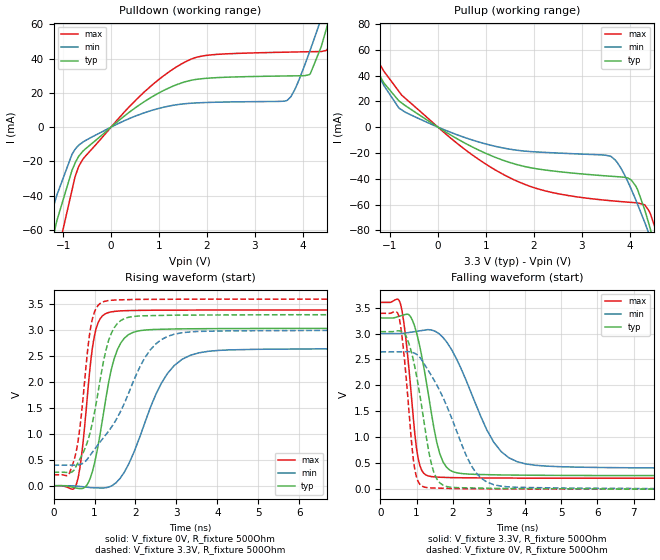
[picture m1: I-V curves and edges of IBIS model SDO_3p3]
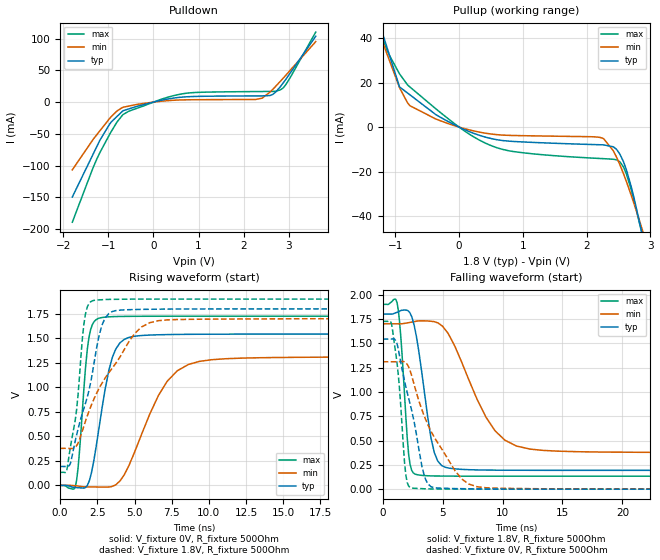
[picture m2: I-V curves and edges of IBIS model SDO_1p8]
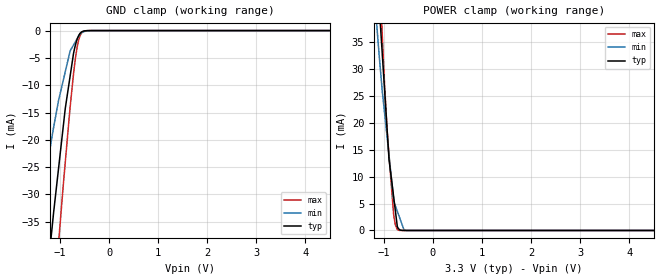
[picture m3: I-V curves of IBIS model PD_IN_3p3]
|Texas Instruments Incorporated
| INTEGRATED POWER AMPLIFIER MONITOR AND CONTROL SYSTEM
| Marketing part#   Digital Voltage Range   Package-type   #pins
| AMC7834   1.7V - 3.6V   PQFP   56
[IBIS Ver]   4.1
[File name]   amc7834.ibs
[File Rev]   1.0
[Date]   12/12/2013
[Source]
| Texas Instruments Incorporated.
| 12500 TI Blvd
| Dallas, TX -75243
[Notes]   Revision History:
| Rev 1.0: 12/12/2013
| - Initial version of the model
| - Model generated from simulations in TISPICE
| - C_comp although listed in numerical order of value are
|   obtained from varying PVT conditions. For PVT conditions for
|   each specific value refer the buffer description under
|   respective [Model]. IBIS model user is responsible for using
|   appropriate C_comp to simulate for Signal Integrity.
| - Model names with a trailing _1p8 contains the model for
|   1.8V operation.Model names with a trailing _3p3 contains the model
|   for 3.3V operation.
[Disclaimer]
| This model is designed as an aid for customers of Texas Instruments.
| TI and its licensors and suppliers make no warranties, either expressed
| or implied, with respect to this  model, including the warranties of
| merchantability or fitness for a particular purpose. The model is
| provided solely on an "as is" basis. The entire risk as to its quality
| and performance is with the customer.
[Copyright]
 (C) Copyright 2013 Texas Instruments Incorporated.All rights reserved.
|   Device
[Component]   AMC7834
[Manufacturer]   TI
[Package]
| variable   typ   min   max
R_pkg   0.079   0.031   0.106
L_pkg   1.073nH   0.648nH   1.372nH
C_pkg   0.150pF   0.128pF   0.230pF
[Pin]  signal_name   model_name   R_pin   L_pin   C_pin
1   DIGTEST/DAV   DAV   0.1053   1.37016nH   0.14918pF
2   ALARMOUT   GPIO   0.09756   1.25753nH   0.14389pF
3   SLEEP1   PD_IN   0.09216   1.17804nH   0.13837pF
4   SLEEP2   PD_IN   0.08922   1.13506nH   0.13484pF
5   RESETB   PD_IN   0.08788   1.1154nH   0.1331pF
6   DACTRIGB   PD_IN   0.08783   1.11459nH   0.13297pF
7   SCLK   PD_IN   0.08841   1.12318nH   0.13416pF
8   CSB   PD_IN   0.09063   1.15576nH   0.13641pF
9   SDI   PD_IN   0.09435   1.21049nH   0.1403pF
10   SDO   SDO   0.09971   1.28996nH   0.14738pF
11   DGND   GND   0.05243   0.93873nH   0.20017pF
12   IOVDD   POWER   0.03437   0.8265nH   0.22739pF
13   DVDD   POWER   0.03123   0.7166nH   0.21314pF
14   AVCC   POWER   0.04716   0.85425nH   0.17448pF
15   AUXDAC1   NC   0.10508   1.3668nH   0.15013pF
16   AUXDAC2   NC   0.09226   1.17816nH   0.1419pF
17   AGND1   GND   0.04621   0.74677nH   0.18488pF
18   AUXDACC3   NC   0.09212   1.1763nH   0.13877pF
19   AUXDACC4   NC   0.08893   1.12891nH   0.13535pF
20   REFIN   NC   0.08344   1.04761nH   0.13155pF
21   REFOUT   NC   0.07963   0.99042nH   0.12761pF
22   AGND2   GND   0.04047   0.64779nH   0.1651pF
23   DAC1   NC   0.08054   1.00265nH   0.1287pF
24   DAC2   NC   0.08248   1.03019nH   0.13198pF
25   AVSS   GND   0.04579   0.82708nH   0.17866pF
26   AVDD1   POWER   0.03183   0.772nH   0.20696pF
27   DAC3   NC   0.09598   1.22739nH   0.14561pF
28   DAC4   NC   0.10574   1.36956nH   0.14859pF
29   VCLAMP2   NC   0.09234   1.17055nH   0.13553pF
30   VCLAMP1   NC   0.08526   1.0683nH   0.13067pF
31   SENSE4-   NC   0.09275   1.179nH   0.13987pF
32   SENSE4+   NC   0.08261   1.02944nH   0.13079pF
33   SENSE3-   NC   0.08268   1.03069nH   0.13044pF
34   SENSE3+   NC   0.08044   0.9979nH   0.12812pF
35   AGND3   GND   0.04051   0.67363nH   0.15767pF
36   SENSE2-   NC   0.08032   0.99598nH   0.12906pF
37   SENSE2+   NC   0.08312   1.03711nH   0.13092pF
38   SENSE1-   NC   0.08304   1.0359nH   0.13159pF
39   SENSE1+   NC   0.0936   1.19177nH   0.14134pF
40   PA_ON   NC   0.09387   1.19554nH   0.14036pF
41   PAVDD   POWER   0.04917   0.87072nH   0.18625pF
42   REF_ADC/CMP   NC   0.0493   0.89668nH   0.17897pF
43   AGND4   GND   0.05376   0.99104nH   0.19612pF
44   AVDD2   POWER   0.03647   0.9263nH   0.23006pF
45   ADC4   NC   0.1057   1.37162nH   0.15535pF
46   ADC3   NC   0.09734   1.24786nH   0.14443pF
47   ADC2   NC   0.09048   1.14719nH   0.13737pF
48   ADC1   NC   0.08561   1.0763nH   0.13075pF
49   D2-   NC   0.09926   1.27608nH   0.14506pF
50   D2+   NC   0.08838   1.11645nH   0.13873pF
51   D1-   NC   0.08306   1.04024nH   0.13298pF
52   D1+   NC   0.08517   1.07249nH   0.13199pF
53   GPIO4   GPIO   0.0862   1.08664nH   0.13088pF
54   GPIO3   GPIO   0.08789   1.11204nH   0.13416pF
55   GPIO2   GPIO   0.09165   1.16832nH   0.13799pF
56   GPIO1   GPIO   0.09825   1.26426nH   0.14243pF
|   Model Selectors
[Model Selector]  SDO
SDO_3p3   SDO buffer in 3.3V power operation
SDO_1p8   SDO buffer in 1.8V power operation
[Model Selector]  PD_IN
PD_IN_3p3   PD_IN buffer in 3.3V power operation
PD_IN_1p8   PD_IN buffer in 1.8V power operation
[Model Selector]  GPIO
GPIO_3p3   GPIO buffer in 3.3V power operation
GPIO_1p8   GPIO buffer in 1.8V power operation
[Model Selector]  DAV
DAV_3p3   DAV buffer in 3.3V power operation
DAV_1p8   DAV buffer in 1.8V power operation
| Models and submodels in the file (8): SDO_3p3 (Output), SDO_1p8 (Output), PD_IN_3p3 (Input), PD_IN_1p8 (Input), GPIO_3p3 (I/O_open_drain), GPIO_1p8 (I/O_open_drain), DAV_3p3 (Output), DAV_1p8 (Output)
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|   Model
[Model]   SDO_3p3
Model_type   Output
Polarity   Non-Inverting
Vmeas = 1.65
Vref = 0
Cref = 1pF
Rref = 100000
|   typ   min   max
C_comp   3.353pF   3.015pF   3.780pF
[Voltage Range]   3.3   3   3.6
[Temperature Range]   27   125   -40
[Pullup Reference]   3.3   3   3.6
[Pulldown Reference]   0   0   0
[Power Clamp Reference]   3.3   3   3.6
[GND Clamp Reference]   0   0   0
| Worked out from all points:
|   slope of the pulldown table from 0 to 0.495 V, typ, clamps not added: 44.7 ohm
|   slope of the pullup table from 0 to 0.495 V, typ, clamps not added: 45 ohm
|   falling waveform, V_fixture 3.3V, R_fixture 500Ohm: 20-80 % time 466ps typ, 998ps min, 281ps max; typ from 3.3 V to 0.259 V
|   rising waveform, V_fixture 0V, R_fixture 500Ohm: 20-80 % time 426ps typ, 846ps min, 261ps max; typ from 0 V to 3.04 V
|   rising waveform, V_fixture 3.3V, R_fixture 500Ohm: 20-80 % time 470ps typ, 1.03ns min, 277ps max; typ from 0.259 V to 3.3 V
|   falling waveform, V_fixture 0V, R_fixture 500Ohm: 20-80 % time 444ps typ, 987ps min, 260ps max; typ from 3.04 V to 0 V
[Pulldown]
|   Voltage   I(typ)   I(min)   I(max)
-3.3V     -387.4mA   -282.5mA   -481.1mA
-1.359V   -84.44mA   -61.69mA   -110.2mA
-1.132V   -54.73mA   -39.76mA   -75.64mA
-587.4mV  -14.03mA   -8.722mA   -18.7mA
699.6mV   15.01mA    8.431mA    20.7mA
1.67V     27.34mA    13.96mA    39.69mA
3.679V    29.87mA    15.75mA    43.76mA
4.155V    31.16mA    45.12mA    44.01mA
4.382V    46.96mA    63.3mA     44.14mA
4.491V    57.51mA    72.21mA    44.78mA
4.66V     74.83mA    85.86mA    51.94mA
6.6V      230.9mA    199.7mA    255.5mA
[Pullup]
|   Voltage   I(typ)   I(min)   I(max)
-3.3V     202.9mA    173.1mA    233.4mA
-1.983V   113.5mA    96.85mA    130.9mA
-1.32V    49.67mA    46.79mA    56.45mA
-815.1mV  20.37mA    14.83mA    27.72mA
561mV     -12.35mA   -8.066mA   -17.25mA
1.67V     -29.24mA   -18mA      -42.19mA
3.61V     -38.05mA   -22.74mA   -57.03mA
4.036V    -41.17mA   -48.52mA   -58.32mA
4.165V    -48.59mA   -59.92mA   -58.68mA
4.402V    -75.41mA   -82.71mA   -64.92mA
4.62V     -105.4mA   -105mA     -88.11mA
6.6V      -415.8mA   -337.5mA   -459.7mA
[Ramp]
R_load = 500
|   typ   min   max
dV/dt_r   1.82193/4.26202e-10   1.58772/8.45992e-10   2.03399/2.61394e-10
dV/dt_f   1.82452/4.66143e-10   1.56168/9.97954e-10   2.0337/2.81346e-10
[Falling Waveform]
V_fixture = 3.3V
V_fixture_min = 3V
V_fixture_max = 3.6V
R_fixture = 500Ohm
C_fixture = 0F
|   Time   V(typ)   V(min)   V(max)
0s        3.3V       3V         3.6V
552.8ps   3.339V     3V         3.578V
715.4ps   3.37V      3.012V     2.83V
1.04ns    2.903V     3.046V     607.4mV
1.402ns   1.502V     3.069V     243.7mV
1.639ns   691mV      2.985V     230.1mV
1.924ns   364.5mV    2.739V     223.6mV
3.138ns   276.9mV    901mV      215.5mV
4.285ns   268.1mV    460.4mV    211.9mV
30ns      259.1mV    397.2mV    210.5mV
[Rising Waveform]
V_fixture = 0V
V_fixture_min = 0V
V_fixture_max = 0V
R_fixture = 500Ohm
C_fixture = 0F
|   Time   V(typ)   V(min)   V(max)
0s        1.789uV    -13.04uV   30.69nV
552.8ps   -44.58mV   -7.67mV    17.38mV
678.8ps   -55.19mV   -16.29mV   548.3mV
853.6ps   66.54mV    -31.83mV   1.968V
1.089ns   786.4mV    -42.12mV   3.148V
1.504ns   2.503V     44.93mV    3.364V
1.924ns   2.952V     578.6mV    3.379V
2.781ns   3.02V      2.166V     3.386V
3.78ns    3.029V     2.593V     3.388V
30ns      3.037V     2.646V     3.39V
[Rising Waveform]
V_fixture = 3.3V
V_fixture_min = 3V
V_fixture_max = 3.6V
R_fixture = 500Ohm
C_fixture = 0F
|   Time   V(typ)   V(min)   V(max)
0s        259.1mV    397.2mV    210.5mV
361.1ps   253.7mV    396.2mV    207.4mV
501ps     301.9mV    395.9mV    491.7mV
641.6ps   511.5mV    411.7mV    1.109V
913.5ps   1.094V     608.5mV    3.086V
1.323ns   2.741V     1.031V     3.569V
1.639ns   3.185V     1.44V      3.585V
2.361ns   3.28V      2.621V     3.594V
3.343ns   3.291V     2.967V     3.598V
30ns      3.3V       3V         3.6V
[Falling Waveform]
|Gnd
V_fixture = 0V
V_fixture_min = 0V
V_fixture_max = 0V
R_fixture = 500Ohm
C_fixture = 0F
|   Time   V(typ)   V(min)   V(max)
0s        3.037V     2.646V     3.39V
522ps     3.051V     2.646V     3.302V
709.1ps   2.95V      2.65V      2.175V
952.5ps   2.353V     2.617V     374.9mV
1.258ns   1.062V     2.362V     33.78mV
1.477ns   326.5mV    2.11V      22.23mV
1.728ns   78.19mV    1.772V     17.54mV
2.633ns   22.58mV    326.8mV    7.131mV
3.343ns   13.16mV    56.94mV    4.511mV
30ns      -7.045uV   -43.35uV   1.992uV
|   Model
[Model]   SDO_1p8
Model_type   Output
Polarity   Non-Inverting
Vmeas = 0.9
Vref = 0
Cref = 1pF
Rref = 100000
|   typ   min   max
C_comp   3.353pF   3.015pF   3.780pF
[Voltage Range]   1.8   1.7   1.9
[Temperature Range]   27   125   -40
[Pullup Reference]   1.8   1.7   1.9
[Pulldown Reference]   0   0   0
[Power Clamp Reference]   1.8   1.7   1.9
[GND Clamp Reference]   0   0   0
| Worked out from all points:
|   slope of the pulldown table from 0 to 0.27 V, typ, clamps not added: 62.8 ohm
|   slope of the pullup table from 0 to 0.27 V, typ, clamps not added: 84.2 ohm
|   falling waveform, V_fixture 1.8V, R_fixture 500Ohm: 20-80 % time 1.12ns typ, 3.01ns min, 552ps max; typ from 1.8 V to 0.193 V
|   rising waveform, V_fixture 0V, R_fixture 500Ohm: 20-80 % time 1.06ns typ, 2.35ns min, 521ps max; typ from 0 V to 1.54 V
|   rising waveform, V_fixture 1.8V, R_fixture 500Ohm: 20-80 % time 1.44ns typ, 2.83ns min, 728ps max; typ from 0.193 V to 1.8 V
|   falling waveform, V_fixture 0V, R_fixture 500Ohm: 20-80 % time 1.55ns typ, 2.99ns min, 674ps max; typ from 1.54 V to 0 V
[Pulldown]
|   Voltage   I(typ)   I(min)   I(max)
-1.8V     -149.4mA   -106.6mA   -189.1mA
-1.253V   -69.45mA   -50.99mA   -89.04mA
-968.4mV  -34.24mA   -25.34mA   -50.26mA
-676.8mV  -13.58mA   -8.132mA   -19.64mA
138.6mV   2.371mA    1.157mA    3.669mA
624.6mV   7.831mA    3.474mA    12.86mA
2.266V    9.809mA    4.161mA    16.64mA
2.412V    9.853mA    6.234mA    16.72mA
2.585V    10.44mA    15.82mA    16.81mA
2.812V    24.04mA    32.53mA    19.24mA
3.044V    46.83mA    50.98mA    39.88mA
3.6V      103.8mA    95.32mA    110.3mA
[Pullup]
|   Voltage   I(typ)   I(min)   I(max)
-1.8V     96.15mA    84.46mA    109.9mA
-1.253V   46.77mA    42.27mA    44.61mA
-1.13V    35.62mA    32.74mA    34.25mA
-936mV    18.11mA    17.78mA    23.96mA
-774mV    14.56mA    9.658mA    18.09mA
-142.2mV  2.055mA    1.303mA    3.109mA
538.2mV   -5.36mA    -3.219mA   -8.715mA
2.25V     -7.964mA   -4.992mA   -14.16mA
2.461V    -9.805mA   -13.04mA   -14.68mA
2.574V    -15.35mA   -20.71mA   -17.78mA
2.866V    -47.46mA   -45.48mA   -47.74mA
3.6V      -154.8mA   -121mA     -178.4mA
[Ramp]
R_load = 500
|   typ   min   max
dV/dt_r   0.925714/1.05755e-09   0.785951/2.34867e-09   1.0351/5.20789e-10
dV/dt_f   0.963998/1.11885e-09   0.793557/3.00656e-09   1.06009/5.52405e-10
[Falling Waveform]
V_fixture = 1.8V
V_fixture_min = 1.7V
V_fixture_max = 1.9V
R_fixture = 500Ohm
C_fixture = 0F
|   Time   V(typ)   V(min)   V(max)
0s        1.8V       1.7V       1.9V
1.205ns   1.818V     1.7V       1.913V
1.497ns   1.836V     1.7V       1.591V
2.167ns   1.828V     1.712V     356.7mV
2.698ns   1.641V     1.724V     155mV
4.024ns   530mV      1.726V     136.5mV
5.221ns   224.9mV    1.639V     134.4mV
8.628ns   196.4mV    738.1mV    133.3mV
11.17ns   194.4mV    443.2mV    133.1mV
30ns      193.3mV    377.4mV    133.2mV
[Rising Waveform]
V_fixture = 0V
V_fixture_min = 0V
V_fixture_max = 0V
R_fixture = 500Ohm
C_fixture = 0F
|   Time   V(typ)   V(min)   V(max)
0s        1.092uV    -18.34uV   218.8nV
1.03ns    -21.66mV   -3.949mV   -6.16mV
1.205ns   -23.25mV   -6.78mV    178mV
1.826ns   -1.261mV   -15.59mV   1.389V
2.556ns   528.5mV    -16.43mV   1.702V
3.273ns   1.173V     -15.99mV   1.719V
4.024ns   1.454V     45.31mV    1.723V
6.609ns   1.536V     916.4mV    1.725V
8.628ns   1.54V      1.233V     1.725V
30ns      1.543V     1.31V      1.725V
[Rising Waveform]
V_fixture = 1.8V
V_fixture_min = 1.7V
V_fixture_max = 1.9V
R_fixture = 500Ohm
C_fixture = 0F
|   Time   V(typ)   V(min)   V(max)
0s        193.3mV    377.6mV    133.2mV
446.2ps   192.5mV    377.5mV    153.3mV
1.106ns   512.9mV    405.7mV    771.7mV
1.591ns   783.3mV    601.8mV    1.639V
2.167ns   1.147V     843.6mV    1.882V
2.624ns   1.532V     990.2mV    1.892V
3.273ns   1.752V     1.149V     1.897V
4.987ns   1.793V     1.544V     1.899V
6.609ns   1.797V     1.68V      1.899V
30ns      1.8V       1.7V       1.9V
[Falling Waveform]
|Gnd
V_fixture = 0V
V_fixture_min = 0V
V_fixture_max = 0V
R_fixture = 500Ohm
C_fixture = 0F
|   Time   V(typ)   V(min)   V(max)
0s        1.543V     1.31V      1.725V
784.4ps   1.544V     1.31V      1.669V
1.302ns   1.44V      1.31V      1.176V
1.937ns   1.049V     1.298V     140.5mV
2.284ns   876mV      1.219V     17.29mV
3.273ns   234mV      816.7mV    5.29mV
3.74ns    59.3mV     670.8mV    3.086mV
6.02ns    5.938mV    192.1mV    676.1uV
7.191ns   3.806mV    52.09mV    643.2uV
30ns      -5.695uV   -47.89uV   1.068uV
|   Model
[Model]   PD_IN_3p3
Model_type   Input
Vinl = 0.99
Vinh = 2.31
|   typ   min   max
C_comp   9.202pF   6.403pF   9.427pF
[Voltage Range]   3.3   3   3.6
[Temperature Range]   27   125   -40
[Power Clamp Reference]   3.3   3   3.6
[GND Clamp Reference]   0   0   0
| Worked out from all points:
|   GND clamp passes 1 mA (typ) near -0.63 V on its own axis
|   POWER clamp passes 1 mA (typ) near -0.73 V on its own axis
[GND Clamp]
|   Voltage   I(typ)   I(min)   I(max)
-3.3V     -260.9mA   -178.9mA   -317.8mA
-1.478V   -65.8mA    -37.74mA   -91.86mA
-1.379V   -56.03mA   -31.72mA   -79.83mA
-1.201V   -39.43mA   -21.39mA   -58.55mA
-1.162V   -35.92mA   -19.27mA   -53.92mA
-1.033V   -25.35mA   -12.85mA   -39.04mA
-894.3mV  -14.24mA   -7.523mA   -24.09mA
-795.3mV  -8.319mA   -3.717mA   -14.01mA
-706.2mV  -3.342mA   -2.335mA   -6.38mA
-627mV    -1.023mA   -1.106mA   -1.95mA
-537.9mV  -146.2uA   -265.3uA   -231.6uA
6.6V      0A         0A         0A
[POWER Clamp]
|   Voltage   I(typ)   I(min)   I(max)
-3.3V     595.2mA    507.8mA    665.1mA
-1.191V   58.76mA    44.15mA    74.63mA
-1.132V   46.91mA    36.66mA    59.8mA
-1.073V   38.47mA    30.07mA    44.97mA
-1.033V   32.85mA    25.91mA    36.34mA
-933.9mV  18.79mA    17.34mA    18.55mA
-894.3mV  13.16mA    13.91mA    13.91mA
-803.7mV  6.489mA    6.066mA    3.29mA
-765.6mV  3.679mA    4.582mA    1.05mA
-706.2mV  397.1uA    3.075mA    78.84uA
-537.9mV  623.1nA    14.62uA    0A
6.6V      0A         0A         0A
